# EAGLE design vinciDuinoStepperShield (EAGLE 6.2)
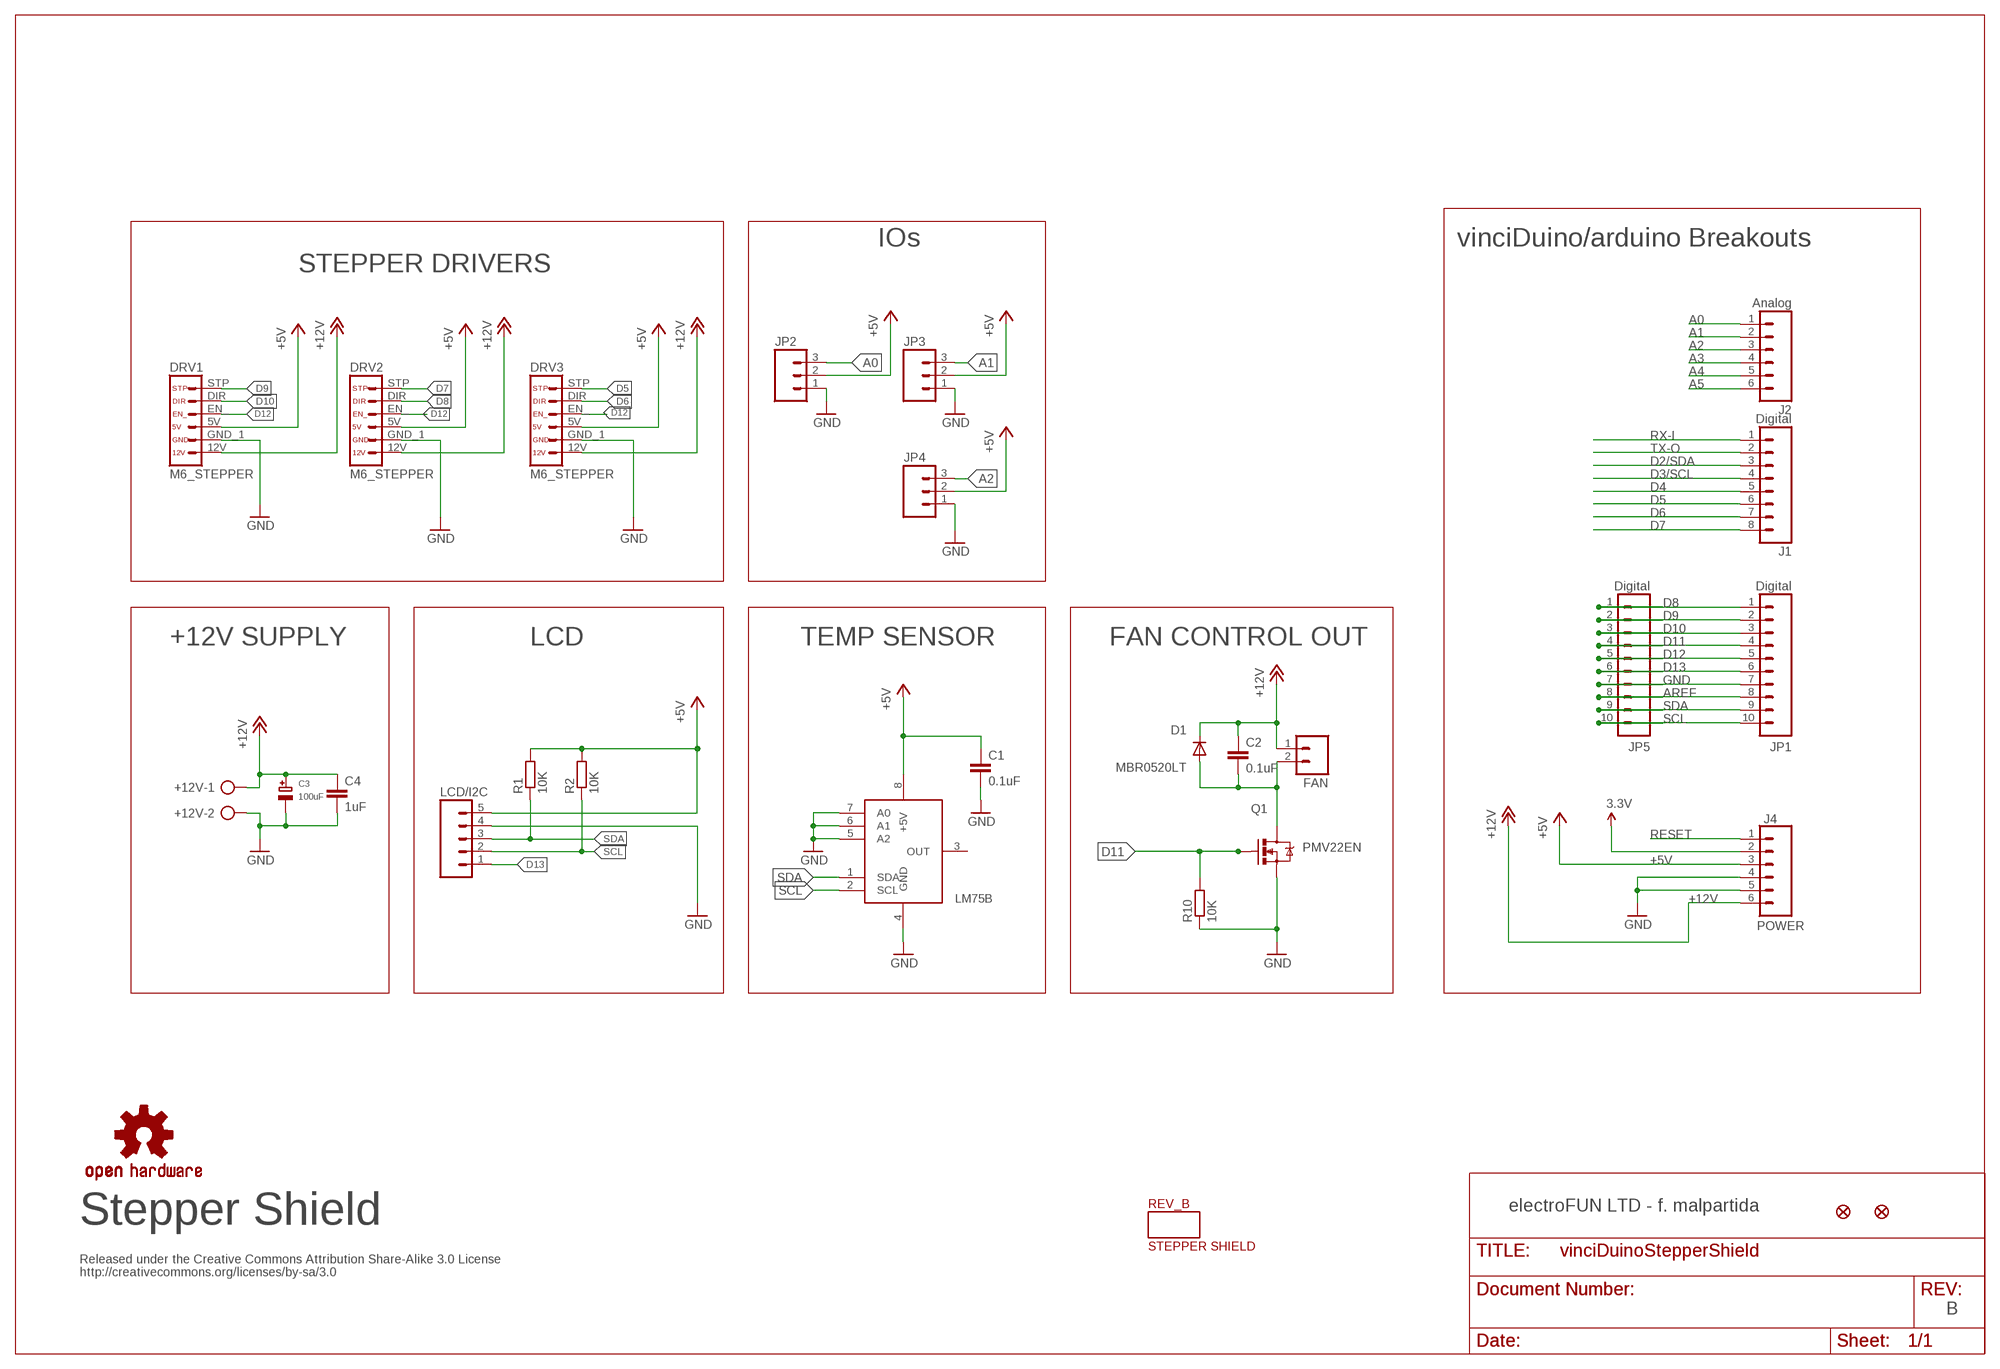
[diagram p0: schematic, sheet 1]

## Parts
+12V  AK500/2  [AK500/2]
C1  0.1uF  C-EUC0805  [C0805]
C2  0.1uF  C-EUC0805  [C0805]
C3  100uF  CAP_ELECTROLYTICPANASONIC_D  [PANASONIC_D]
C4  1uF  C-EUC1206  [C1206]
D1  MBR0520LT  [SOD123]
DRV1  M6_STEPPER  [1X06-STEPPER]
DRV2  M6_STEPPER  [1X06-STEPPER]
DRV3  M6_STEPPER  [1X06-STEPPER]
FAN  M02PTH  [1X02]
IC1  LM75  [SO8]
J1  Digital  M081X08  [1X08]
J2  Analog  M06SIP  [1X06]
J4  POWER  M06SIP  [1X06]
JP1  Digital  M10"  [1X10]
JP2  M03PTH  [1X03]
JP3  M03PTH  [1X03]
JP4  M03PTH  [1X03]
JP5  Digital  M10"  [1X10]
LCD/I2C  M05PTH  [1X05]
Q1  PMV22EN  MOSFET-NCHANNELSMD  [SOT23-3]
R1  10K  R-EU_R0805  [R0805]
R2  10K  R-EU_R0805  [R0805]
R10  10K  R-EU_R0805  [R0805]
REV_B  STEPPER SHIELD  BOARD_INFOL+  [BOARD_INFO_LARGE]
U$2  FIDUCIAL1X2  [FIDUCIAL-1X2]
U$4  FIDUCIAL1X2  [FIDUCIAL-1X2]
U$6  OSHW-LOGOM  [OSHW-LOGO-M]

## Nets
3.3V: J4.2
+5V [power]: C1.1 DRV1.5V DRV2.5V DRV3.5V IC1.8(+5V) J4.3 JP2.2 JP3.2 JP4.2 LCD/I2C.5 R1.2 R2.2
+12V [12V]: +12V.1 C2.1 C3.+ C4.1 D1.C DRV1.12V DRV2.12V DRV3.12V FAN.1 J4.6
A0: J2.1 JP2.3
A1: J2.2 JP3.3
A2: J2.3 JP4.3
A3: J2.4
A4: J2.5
A5: J2.6
AREF: JP1.8 JP5.8
D2/SDA: J1.3
D3/SCL: J1.4
D4: J1.5
D5: DRV3.STP J1.6
D6: DRV3.DIR J1.7
D7: DRV2.STP J1.8
D8: DRV2.DIR JP1.1 JP5.1
D9: DRV1.STP JP1.2 JP5.2
D10: DRV1.DIR JP1.3 JP5.3
D11: JP1.4 JP5.4 Q1.1(G) R10.2
D12: DRV1.EN_ DRV2.EN_ DRV3.EN_ JP1.5 JP5.5
D13: JP1.6 JP5.6 LCD/I2C.1
GND: +12V.2 C1.2 C3.- C4.2 DRV1.GND_1(GND) DRV2.GND_1(GND) DRV3.GND_1(GND) IC1.4(GND) IC1.5(A2) IC1.6(A1) IC1.7(A0) J4.4 J4.5 JP1.7 JP2.1 JP3.1 JP4.1 JP5.7 LCD/I2C.4 Q1.2(S) R10.1
N$7 [power]: C2.2 D1.A FAN.2 Q1.3(D)
RESET: J4.1
RX-I: J1.1
SCL: IC1.2(SCL) JP1.10 JP5.10 LCD/I2C.2 R2.1
SDA: IC1.1(SDA) JP1.9 JP5.9 LCD/I2C.3 R1.1
TX-O: J1.2
Unconnected: IC1.3(OUT)

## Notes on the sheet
- IOs | vinciDuino/arduino Breakouts
- STEPPER DRIVERS
- +12V SUPPLY | LCD | TEMP SENSOR | FAN CONTROL OUT
- LM75B
- electroFUN LTD - f. malpartida
- Stepper Shield
- Released under the Creative Commons Attribution Share-Alike 3.0 License
- http://creativecommons.org/licenses/by-sa/3.0
- B

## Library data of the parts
+12V = con-ptr500:AK500/2: CONNECTOR; OC_FARNELL: unknown; OC_NEWARK: unknown
C1 C2 C4 = rcl:C-EU: CAPACITOR, European symbol
C3 = microbuilder:CAP_ELECTROLYTIC: Electrolytic Capacitors
D1 = diode:MBR0520LT: SCHOTTKY BARRIER RECTIFIER
DRV1-DRV3 = SparkFun:M6_STEPPER
FAN = SparkFun:M02: Header 2
IC1 = lm75:LM75
J1 = SparkFun:M08: Header 8 Standard 8-pin 0.1" header. Use with straight break away headers (SKU : PRT-00116), right angle break away headers (PRT-00553), swiss pins (PRT-00743), machine pins (PRT-00117), and female headers (PRT-00115).
J2 J4 = SparkFun:M06: Header 6 Standard 6-pin 0.1" header. Use with straight break away headers (SKU : PRT-00116), right angle break away headers (PRT-00553), swiss pins (PRT-00743), machine pins (PRT-00117), and female headers (PRT-00115). Molex polarized connector foot print use with SKU : PRT-08094 with associated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
JP1 JP5 = SparkFun:M10: Header 10 Standard 10-pin 0.1" header. Use with straight break away headers (SKU : PRT-00116), right angle break away headers (PRT-00553), swiss pins (PRT-00743), machine pins (PRT-00117), and female headers (PRT-00115).
JP2-JP4 = SparkFun:M03: Header 3 Standard 3-pin 0.1" header. Use with straight break away headers (SKU : PRT-00116), right angle break away headers (PRT-00553), swiss pins (PRT-00743), machine pins (PRT-00117), and female headers (PRT-00115). Molex polarized connector foot print use with SKU : PRT-08232 with associated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
LCD/I2C = SparkFun:M05: Header 5 Standard 5-pin 0.1" header. Use with straight break away headers (SKU : PRT-00116), right angle break away headers (PRT-00553), swiss pins (PRT-00743), machine pins (PRT-00117), and female headers (PRT-00115). Molex polarized connector foot print use with SKU : PRT-08230 with associated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
Q1 = SparkFun:MOSFET-NCHANNEL
R1 R2 R10 = resistor:R-EU_: RESISTOR, European symbol
REV_B = fmc:BOARD_INFO
U$2 U$4 = SparkFun:FIDUCIAL: Fiducial Alignment Points
U$6 = SparkFun:OSHW-LOGO: Open Source Hardware Logo This logo indicates the piece of hardware it is found on incorporates a OSHW license and/or adheres to the definition of open source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

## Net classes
0 default: width 0.152 mm, clearance 0.152 mm
1 power: width 0.508 mm, clearance 0.305 mm
2 12V: width 1 mm, clearance 0.406 mm

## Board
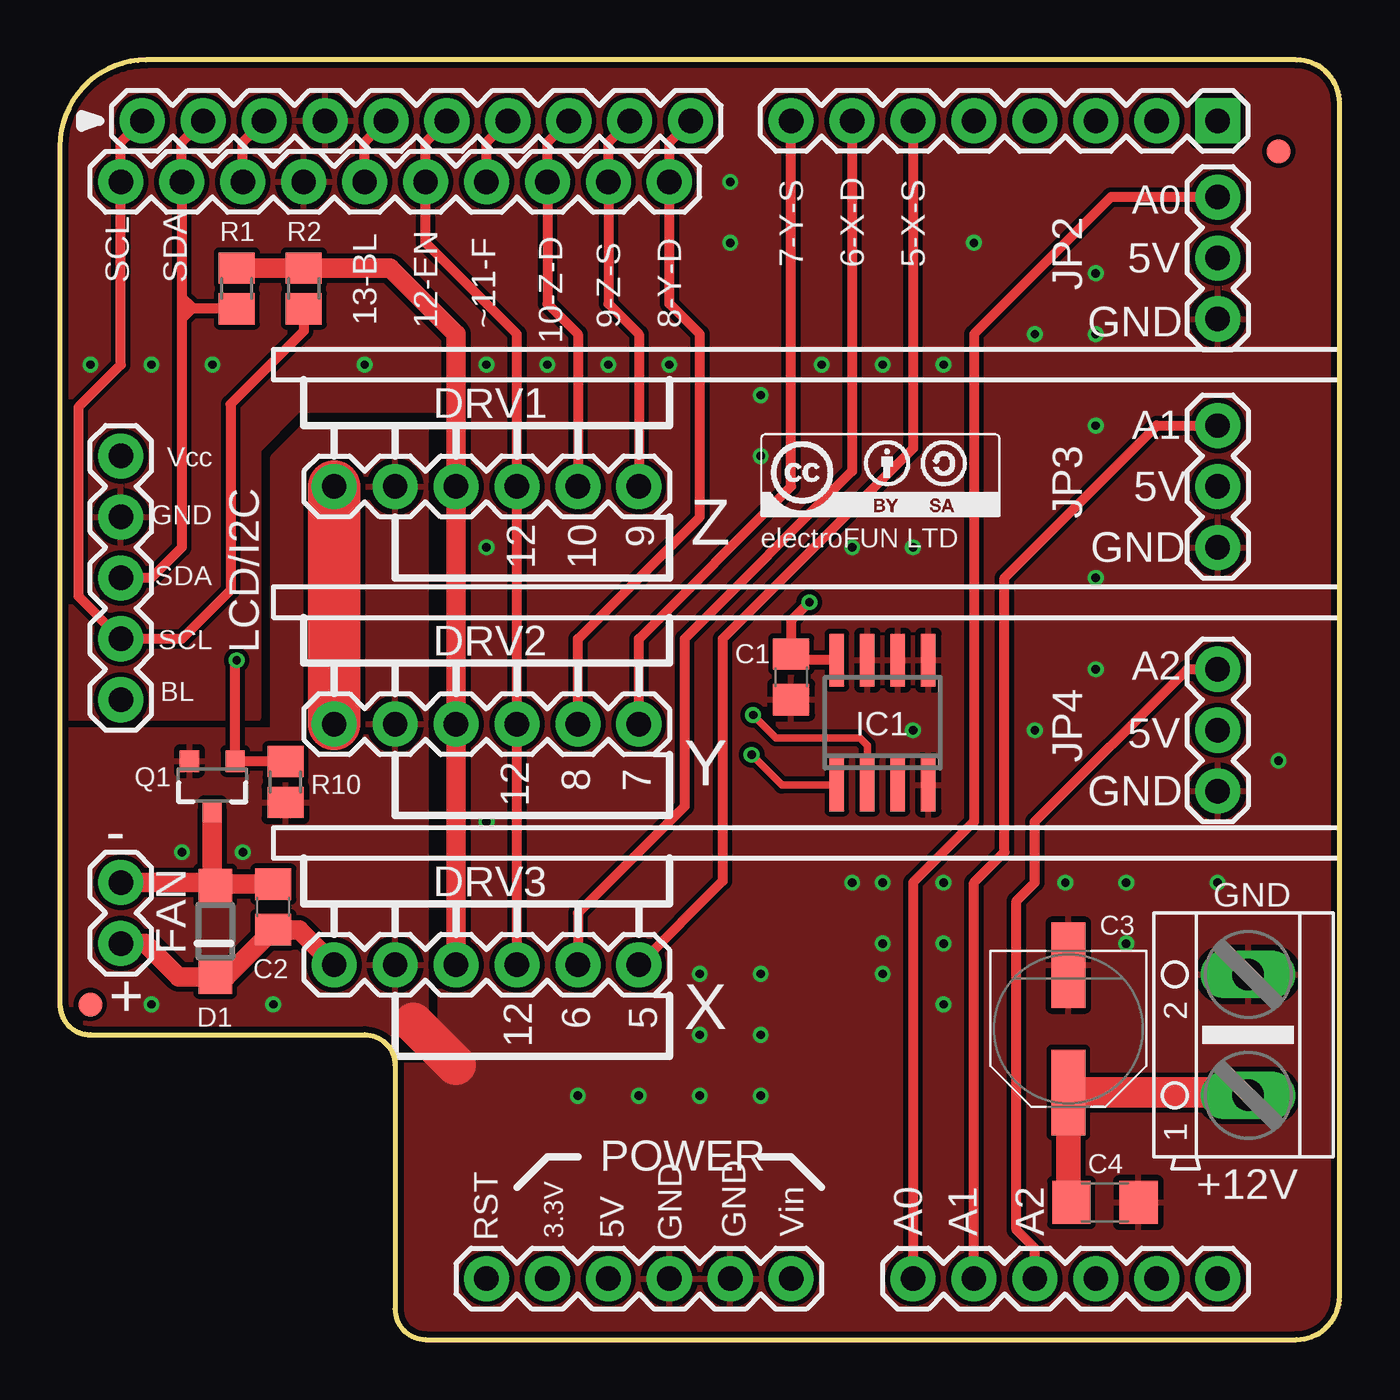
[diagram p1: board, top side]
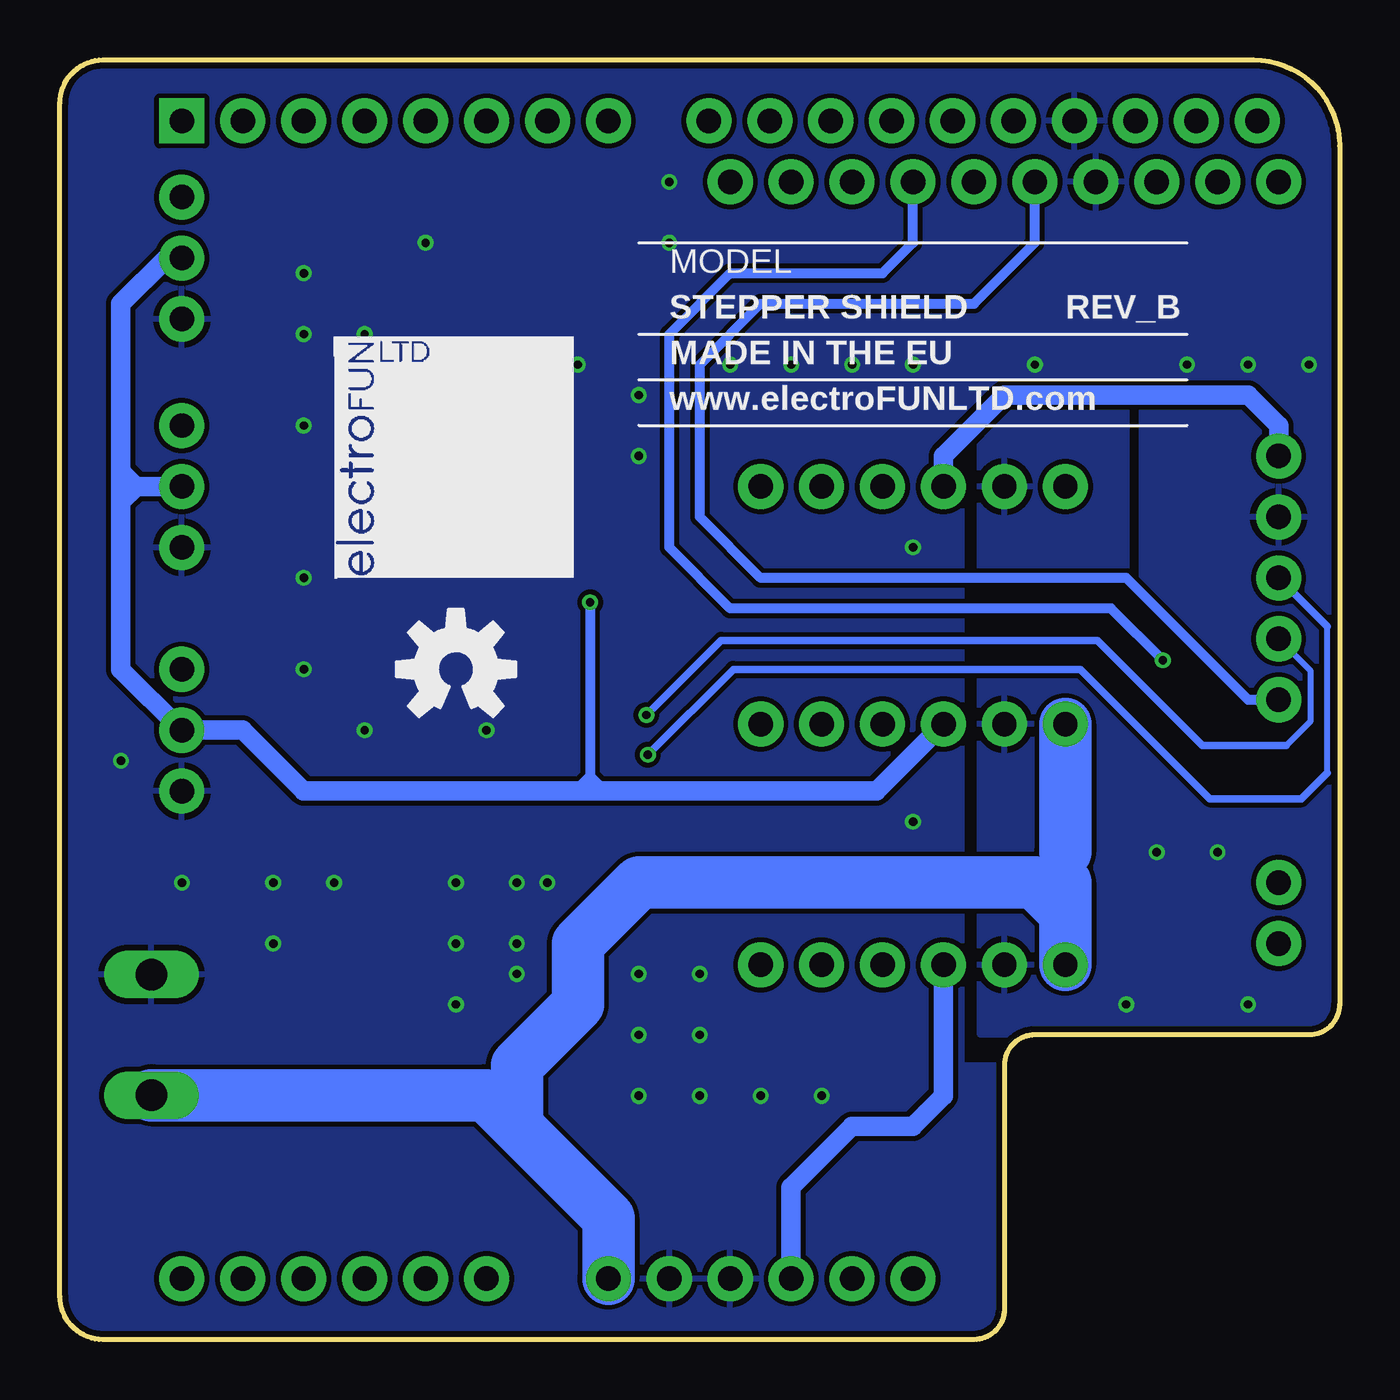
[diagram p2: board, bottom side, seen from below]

Size 53.34 x 53.34 mm. Coordinates in mm from the lower left corner, seen from the top.
Outline: 53.34,51.54 arc90 51.54,53.34 3.59,53.34 arc90 0,49.75 0,13.97 arc90 1.27,12.7 12.7,12.7 arc-90 13.97,11.43 13.97,1.27 arc90 15.24,0 51.54,0 arc90 53.34,1.8 53.34,51.54
Copper layers (1*16): Top 0.0356mm / dielectric 1.5011mm / Bottom 0.0356mm
Design rules: minimum track width 6mil, minimum drill 0.35mm, track to track 8mil, track to pad 8mil, pad to pad 8mil, via to via 8mil, smd to smd 8mil, copper to edge 10mil, drill to drill 6mil, minimum pad ring 12mil, minimum via ring 6mil, stop-mask expansion 4mil, vias tented up to drill 25mil, thermal gap 10mil

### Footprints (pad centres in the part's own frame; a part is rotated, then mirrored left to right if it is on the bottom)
AK500/2 = drill 1.321 long: 1 -2.515,0; 2 2.515,0
C0805 = smd 1.3 x 1.5: 1 -0.95,0; 2 0.95,0
PANASONIC_D = smd 3.556 x 1.4: + 2.654,0; - -2.654,0
C1206 = smd 1.6 x 1.8: 1 -1.4,0; 2 1.4,0
SOD123 = smd 1.4 x 1.4: A 1.9,0; C -1.9,0
1X06-STEPPER = drill 1.016 pad 1.88: 5V 5.08,0; 12V 0,0; DIR 10.16,0; EN_ 7.62,0; GND_1 2.54,0; STP 12.7,0
1X02 = drill 1.016 pad 1.88: 1 0,0; 2 2.54,0
SO8 = smd 0.6 x 2.2: 1 -1.905,-2.6; 2 -0.635,-2.6; 3 0.635,-2.6; 4 1.905,-2.6; 5 1.905,2.6; 6 0.635,2.6; 7 -0.635,2.6; 8 -1.905,2.6
1X08@1 = drill 1.016 pad 1.88 square: 1 0,0 | drill 1.016 pad 1.88: 2 2.54,0; 3 5.08,0; 4 7.62,0; 5 10.16,0; 6 12.7,0; 7 15.24,0; 8 17.78,0
1X06@1 = drill 1.016 pad 1.88: 1 -6.35,0; 2 -3.81,0; 3 -1.27,0; 4 1.27,0; 5 3.81,0; 6 6.35,0
1X10 = drill 1.016 pad 1.88: 1 0,0; 2 2.54,0; 3 5.08,0; 4 7.62,0; 5 10.16,0; 6 12.7,0; 7 15.24,0; 8 17.78,0; 9 20.32,0; 10 22.86,0
1X03 = drill 1.016 pad 1.88: 1 0,0; 2 2.54,0; 3 5.08,0
1X05 = drill 1.016 pad 1.88: 1 0,0; 2 2.54,0; 3 5.08,0; 4 7.62,0; 5 10.16,0
SOT23-3 = smd 0.8 x 0.9: 1 -0.95,-1; 2 0.95,-1; 3 0,1.1
R0805 = smd 1.3 x 1.5: 1 -0.85,0; 2 0.85,0
FIDUCIAL-1X2 = smd 1 x 1: 1 0,0

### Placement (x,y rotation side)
+12V  49.53,12.7 90 top
C1  30.48,27.62 270 top
C2  8.89,18.03 90 top
C3  42.04,12.95 270 top
C4  43.56,5.71 0 top
D1  6.48,17.02 90 top
DRV1  11.43,35.56 0 top
DRV2  11.43,25.65 0 top
DRV3  11.43,15.62 0 top
FAN  2.54,16.51 90 top
IC1  34.29,25.72 0 top
J1  Digital  [1X08@1]  48.26,50.8 180 top
J2  Analog  [1X06@1]  41.91,2.54 0 top
J4  POWER  [1X06@1]  24.13,2.54 0 top
JP1  26.29,50.8 180 top
JP2  48.26,42.55 90 top
JP3  48.26,33.02 90 top
JP4  48.26,22.86 90 top
JP5  25.4,48.26 180 top
LCD/I2C  2.54,26.67 90 top
Q1  6.35,23.11 180 top
R1  7.37,43.81 90 top
R2  10.16,43.81 90 top
R10  9.4,23.24 90 top
REV_B  17.78,39.37 0 bottom
U$1  [ELECTROFUN]  41.91,31.75 0 bottom
U$2  1.27,13.97 0 top
U$4  50.8,49.53 0 top
U$5  [SA-BY]  29.21,34.29 0 top
U$6  36.83,27.94 0 bottom

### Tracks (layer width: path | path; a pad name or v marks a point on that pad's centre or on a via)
+5V  (via drill 0.35)
  Top 0.406: 30.86,28.32 IC1.8 30.73,28.32 C1.1 30.48,29.97 v31.24,30.73
  Top 0.813: R1.2 R2.2 13.76,44.66 16.51,41.91 DRV1.5V DRV2.5V DRV3.5V
  Bottom 0.406: v31.24,30.73 31.24,23.5 | 31.24,23.5 31.24,23.37 31.75,22.86 | 31.24,23.5 30.61,22.86 | 31.24,23.5 31.88,22.86
  Bottom 0.813: J4.3 22.86,6.35 20.32,8.89 17.78,8.89 16.51,10.16 DRV3.5V | DRV1.5V 16.51,36.83 13.97,39.37 3.81,39.37 2.54,38.1 LCD/I2C.5 | 16.51,25.4 DRV2.5V 19.3,22.86 30.61,22.86 31.75,22.86 31.88,22.86 43.18,22.86 45.72,25.4 JP4.2 50.8,27.94 50.8,34.92 | JP2.2 48.9,45.09 50.8,43.18 50.8,36.2 | 50.8,35.56 50.8,34.92 | JP3.2 50.16,35.56 | 50.16,35.56 50.8,35.56 | 50.16,35.56 50.8,36.2 | 50.8,36.2 50.8,35.56 | 50.8,34.92 50.16,35.56
+12V
  Top 0.813: FAN.1 3.56,16.51 4.95,15.12 D1.C 6.92,15.12 C2.1 9.97,17.08 DRV3.12V
  Top 1.016: C3.+ 42.04,5.84 C4.1
  Top 1.27: C3.+ 49.41,10.3 +12V.1
  Top 2.184: DRV1.12V DRV2.12V
  Bottom 1.27: 34.29,11.43 35.53,10.19 35.54,10.19 35.56,10.16 35.59,10.19 | 12.7,19.05 11.43,19.05 11.43,20.32 12.7,19.05
  Bottom 2.184: +12V.1 35.59,10.19 | 11.43,19.05 11.43,17.78 | 11.43,17.78 DRV3.12V | DRV2.12V 11.43,20.32 | 11.43,17.78 12.7,19.05 29.21,19.05 31.75,16.51 31.75,13.97 34.29,11.43 34.29,8.89 | 35.56,10.16 30.48,5.08 J4.6
A0
  Top 0.406: JP2.3 43.81,47.62 38.1,41.91 38.1,21.59 35.56,19.05 J2.1
A1
  Top 0.406: J2.2 38.1,19.05 39.37,20.32 39.37,31.75 45.72,38.1 JP3.3
A2
  Top 0.406: JP4.3 46.99,27.94 40.64,21.59 40.64,19.05 39.88,18.29 39.88,4.57 40.64,3.81 J2.3
AREF
  Top 0.406: JP5.8 7.62,49.91 JP1.8
D5
  Top 0.406: 24.13,15.56 DRV3.STP 27.62,19.11 27.62,29.21 35.56,37.15 J1.6
D6
  Top 0.406: 21.59,15.56 DRV3.DIR 21.59,17.78 26.04,22.23 26.04,29.21 33.02,36.2 J1.7
D7
  Top 0.406: DRV2.STP 24.13,29.21 30.48,35.56 J1.8
D8
  Top 0.406: JP1.1 25.4,49.91 JP5.1 25.4,43.18 26.67,41.91 26.67,34.29 21.59,29.21 DRV2.DIR
D9
  Top 0.406: JP1.2 22.86,49.91 JP5.2 22.86,43.18 24.13,41.91 DRV1.STP
D10
  Top 0.406: JP1.3 20.32,49.91 JP5.3 20.32,43.18 21.59,41.91 DRV1.DIR
D11  (via drill 0.35)
  Top 0.406: JP5.4 17.78,49.91 JP1.4 | R10.2 9.38,24.11 Q1.1 7.3,28.25 v7.37,28.32
  Bottom 0.406: JP5.4 17.78,45.72 19.05,44.45 25.4,44.45 27.94,41.91 27.94,33.02 25.4,30.48 9.53,30.48 v7.37,28.32
D12
  Top 0.406: JP1.5 15.24,49.91 JP5.5 15.24,45.72 19.05,41.91 DRV1.EN_ DRV2.EN_ DRV3.EN_
D13
  Top 0.406: JP5.6 12.7,49.91 JP1.6
  Bottom 0.406: LCD/I2C.1 3.81,26.67 8.89,31.75 24.13,31.75 26.67,34.29 26.67,40.64 24.13,43.18 15.24,43.18 12.7,45.72 JP5.6
GND  (via drill 0.35)
  Top 1.676: 14.73,13.21 16.51,11.43
  other vias: 43.18,38.1 40.64,41.91 43.18,41.91 43.18,44.45 43.18,31.75 43.18,27.94 40.64,25.4 50.8,24.13 44.45,19.05 48.26,19.05 36.83,16.51 36.83,13.97 26.67,12.7 29.21,12.7 29.21,10.16 26.67,10.16 24.13,10.16 26.67,15.24 29.21,15.24 33.02,19.05 34.29,19.05 33.02,33.02 35.56,33.02 38.1,45.72 27.94,45.72 27.94,48.26 29.21,39.37 29.21,36.83 21.59,10.16 8.89,13.97 3.81,13.97 6.35,40.64 12.7,40.64 35.56,25.4 17.78,33.02 17.78,40.64 17.78,21.59 7.62,20.32 5.08,20.32 20.32,40.64 22.86,40.64 25.4,40.64 3.81,40.64 1.27,40.64 31.75,40.64 34.29,40.64 36.83,40.64 41.91,19.05 44.45,16.51 36.83,19.05 34.29,16.51 34.29,15.24
  pour Top: 0,25.91 0,53.34 53.34,53.34 53.34,-0.38 13.84,-0.51 13.84,11.43 15.88,11.43 15.88,38.73 9.91,38.73 8.26,37.08 8.26,25.91
  pour Top: 0,25.4 8.89,25.4 8.89,36.79 10.2,38.1 15.24,38.1 15.24,12.7 0,12.7
  pour Bottom: 0,25.91 0,53.34 53.34,53.34 53.34,-0.64 13.72,-0.64 13.84,11.43 15.75,11.43 15.75,38.73 8.26,38.73 8.26,25.91
  pour Bottom: 0,25.4 0,12.7 14.99,12.7 14.99,38.86 8.89,38.86 8.89,25.4
N$7
  Top 0.813: Q1.3 6.35,19.05 D1.A | FAN.2 6.34,19.05 D1.A | C2.2 6.54,18.98 D1.A
SCL  (via drill 0.35)
  Top 0.305: IC1.2 33.66,24.77 33.34,25.08 29.84,25.08 v28.89,26.04
  Top 0.406: JP1.10 2.54,49.91 JP5.10 2.54,40.64 0.76,38.86 0.76,30.99 LCD/I2C.2 5.08,29.21 7.11,31.24 7.11,38.99 10.16,42.04 R2.1
  Bottom 0.254: 2.22,24.77 1.21,25.78 1.21,27.88 LCD/I2C.2
  Bottom 0.305: 2.22,24.77 5.71,24.77 10.1,29.15 25.78,29.15 v28.89,26.04
SDA  (via drill 0.35)
  Top 0.305: v28.83,24.38 30.1,23.12 IC1.1
  Top 0.406: JP1.9 5.08,49.91 JP5.9 5.08,43.43 | 5.08,43.43 5.08,43.18 | 5.08,43.18 5.08,42.55 | 5.08,42.55 5.08,33.02 3.81,31.75 LCD/I2C.3 | R1.1 5.29,42.97 5.08,43.18 | 5.08,43.43 5.46,43.05 5.46,42.93 5.08,42.55
  Bottom 0.254: 0.51,23.62 0.51,29.72
  Bottom 0.305: 0.51,23.62 1.59,22.54 5.4,22.54 10.79,27.94 25.27,27.94 v28.83,24.38 | 0.51,29.72 LCD/I2C.3

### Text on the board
tPlace: A0 | 5V | 7-Y-S | 6-X-D | 5-X-S | SCL | SDA | GND | 13-BL | 12-EN | ~11-F | 10-Z-D | 9-Z-S | 8-Y-D | A1 | Vcc | 5V | GND | Z | GND | 9 | electroFUN LTD | SDA | 12 | 10 | SCL | A2 | BL | 5V | Y | GND | 8 | 7 | 12 | - | GND | X | + | 6 | 5 | 12 | POWER | RST | 3.3V | 5V | GND | GND | Vin | A0 | A1 | A2
tDocu: Released under the Creative Commons Attribution Share-Alike 3.0 License | http://creativecommons.org/licenses/by-sa/3.0 | stepperShield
